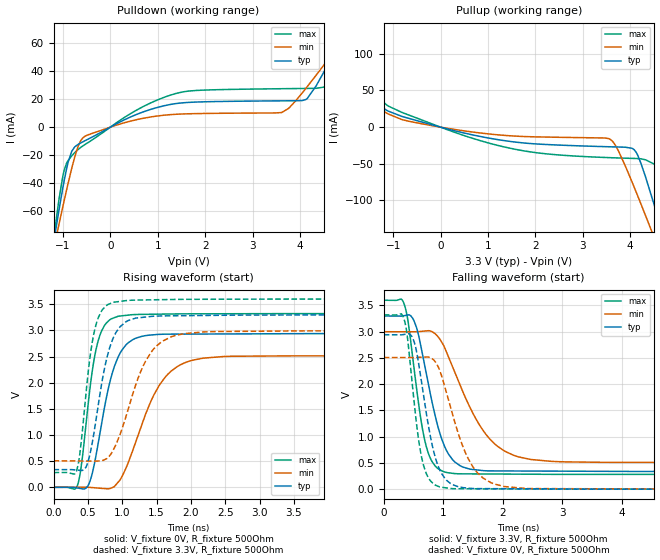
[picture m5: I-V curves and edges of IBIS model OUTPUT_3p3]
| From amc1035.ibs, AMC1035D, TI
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|   OUTPUT_3p3 Model
[Model]   OUTPUT_3p3
Model_type   Output
Polarity   Non-Inverting
Vmeas = 1.65
Vref = 0
Cref = 2pF
Rref = 100000
|   typ   min   max
C_comp   1.505E-12   1.485E-12   1.526E-12
|  Where Nom  PVT is Nominal Process, 3.3V,   27C
|   Fast PVT is Strong Process,  3.6V,   -40C
|   Slow PVT is Weak Process,   3.0V,   131C
[Voltage Range]   3.3   3   3.6
|Junction Temperature
[Temperature Range]   27   131   -40
[Pullup Reference]   3.3   3   3.6
[Pulldown Reference]   0   0   0
[Power Clamp Reference]   3.3   3   3.6
[GND Clamp Reference]   0   0   0
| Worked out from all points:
|   slope of the pulldown table from 0 to 0.495 V, typ, clamps not added: 60 ohm
|   slope of the pullup table from 0 to 0.495 V, typ, clamps not added: 62.2 ohm
|   falling waveform, V_fixture 3.3V, R_fixture 500Ohm: 20-80 % time 356ps typ, 650ps min, 247ps max; typ from 3.3 V to 0.338 V
|   rising waveform, V_fixture 0V, R_fixture 500Ohm: 20-80 % time 283ps typ, 475ps min, 194ps max; typ from 0 V to 2.94 V
|   rising waveform, V_fixture 3.3V, R_fixture 500Ohm: 20-80 % time 253ps typ, 415ps min, 177ps max; typ from 0.338 V to 3.3 V
|   falling waveform, V_fixture 0V, R_fixture 500Ohm: 20-80 % time 278ps typ, 447ps min, 205ps max; typ from 2.94 V to 0 V
[Pulldown]
|   Voltage   I(typ)   I(min)   I(max)
-3.3V     -555.2mA   -439.6mA   -686.6mA
-1.201V   -83.37mA   -87.94mA   -80.92mA
-1.092V   -60.79mA   -70.64mA   -53.34mA
-973.5mV  -37.94mA   -52.26mA   -30.68mA
-815.1mV  -17.19mA   -29.34mA   -20.47mA
-537.9mV  -9.75mA    -6.556mA   -12.48mA
1.363V    16.76mA    9.157mA    23.86mA
3.62V     18.8mA     10.51mA    27.47mA
4.135V    19.91mA    28.06mA    27.67mA
4.511V    39.7mA     44.62mA    28.62mA
4.966V    70.11mA    65.89mA    63.66mA
6.6V      184.6mA    145.6mA    222.9mA
[Pullup]
|   Voltage   I(typ)   I(min)   I(max)
-3.3V     158.9mA    113.8mA    220mA
-2.033V   74.78mA    56.26mA    100.2mA
-1.102V   21.75mA    17.88mA    28.71mA
1.284V    -17.79mA   -10.89mA   -26.09mA
3.551V    -26.74mA   -15.68mA   -41.57mA
3.739V    -27.06mA   -30.5mA    -42mA
4.125V    -33.9mA    -87.93mA   -42.78mA
4.333V    -69.07mA   -121.6mA   -44.68mA
4.511V    -106.3mA   -150.9mA   -50.44mA
4.67V     -140.8mA   -177.3mA   -76.92mA
4.877V    -186.8mA   -212mA     -131.7mA
6.6V      -578mA     -504.2mA   -630.5mA
[Ramp]
R_load = 500
|   typ   min   max
dV/dt_r   1.76545/2.8205e-10   1.50552/4.72282e-10   1.99287/1.94478e-10
dV/dt_f   1.77733/3.54642e-10   1.49559/6.48301e-10   1.99069/2.46584e-10
[Falling Waveform]
V_fixture = 3.3V
V_fixture_min = 3V
V_fixture_max = 3.6V
R_fixture = 500Ohm
C_fixture = 0F
|   Time   V(typ)   V(min)   V(max)
0s        3.3V       3V         3.6V
333.8ps   3.304V     2.999V     3.555V
501ps     3.225V     2.999V     2.377V
634.6ps   2.663V     3.008V     1.253V
764.8ps   1.918V     3.018V     637mV
967.1ps   975.4mV    2.813V     354.1mV
1.194ns   517.8mV    2.226V     296.7mV
1.854ns   347.9mV    871.1mV    288.7mV
2.933ns   343.2mV    524mV      282.4mV
45.47ns   337.8mV    507.3mV    282.2mV
[Rising Waveform]
V_fixture = 0V
V_fixture_min = 0V
V_fixture_max = 0V
R_fixture = 500Ohm
C_fixture = 0F
|   Time   V(typ)   V(min)   V(max)
0s        -48.47nV   -94.48nV   -65.95nV
345.5ps   -12.38mV   310.5uV    28.43mV
511.5ps   53.62mV    459.7uV    1.68V
597.7ps   467.6mV    -8.747mV   2.497V
697.1ps   1.194V     -19.5mV    2.982V
888ps     2.32V      18.45mV    3.245V
1.133ns   2.805V     631.7mV    3.3V
1.666ns   2.929V     2.165V     3.314V
2.583ns   2.933V     2.506V     3.319V
45.47ns   2.942V     2.509V     3.321V
[Rising Waveform]
V_fixture = 3.3V
V_fixture_min = 3V
V_fixture_max = 3.6V
R_fixture = 500Ohm
C_fixture = 0F
|   Time   V(typ)   V(min)   V(max)
0s        337.8mV    507.3mV    282.2mV
333.8ps   330.8mV    504mV      306.6mV
471.6ps   382.3mV    502.6mV    1.778V
560ps     825.9mV    501.7mV    2.747V
654.7ps   1.602V     503.7mV    3.254V
836.3ps   2.745V     638.7mV    3.519V
1.074ns   3.18V      1.438V     3.573V
1.497ns   3.274V     2.7V       3.587V
2.363ns   3.289V     2.979V     3.596V
45.47ns   3.3V       3V         3.6V
[Falling Waveform]
|Gnd
V_fixture = 0V
V_fixture_min = 0V
V_fixture_max = 0V
R_fixture = 500Ohm
C_fixture = 0F
|   Time   V(typ)   V(min)   V(max)
0s        2.942V     2.509V     3.321V
322.4ps   2.944V     2.509V     3.299V
486.2ps   2.878V     2.508V     1.929V
597.7ps   2.313V     2.513V     849.9mV
697.1ps   1.583V     2.517V     350.2mV
888ps     522.4mV    2.387V     66.18mV
1.133ns   101.3mV    1.518V     11.53mV
1.578ns   10.88mV    306.2mV    6.736mV
2.472ns   6.635mV    11.24mV    2.814mV
45.47ns   19.76uV    20.91uV    18.17uV
